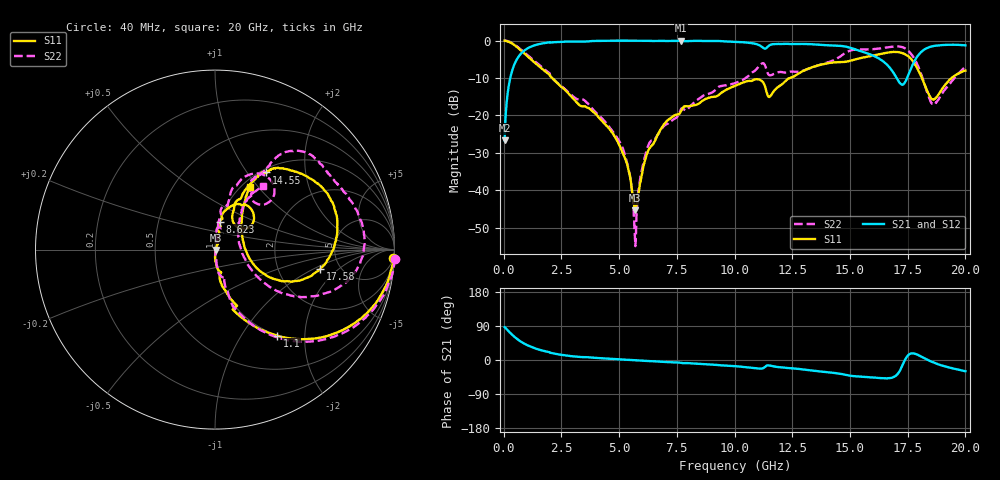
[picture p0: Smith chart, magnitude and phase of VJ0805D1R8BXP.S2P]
! VJ0805D1R8BXP
! DATE 10/29/2021  11:30
! CAPACITORS MOUNTED IN SERIES ON 25 MIL THICK MICROSTRIP SUBSTRATE
# GHz  S  MA  R  50.00
!  FREQ  S11M  S11A  S21M  S21A  S12M  S12A  S22M  S22A
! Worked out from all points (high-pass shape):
!   1601 points, 40 MHz to 20 GHz, reference 50 ohm
!   highest |S21| = 0.00 dB at 7.662 GHz (marker M1); lowest = -26.6 dB at 40 MHz (marker M2)
!   |S21| within 3 dB of the highest: 831 MHz to 15.55 GHz (14.72 GHz wide, 180 % of centre); 18.09 GHz to end of sweep
!   lowest |S11| = -45.3 dB at 5.704 GHz (marker M3), VSWR 1.01, Z = 50.5 - j0.143 ohm
!   |S11| at or under -10 dB: 2.098 GHz to 12.41 GHz (10.31 GHz wide, 142 % of centre); 18.12 GHz to 19.4 GHz (1.282 GHz wide, 6.84 % of centre)
!   |S22| runs from -54.9 to 0.0 dB; largest |S21 - S12| = 0.0054
!   S11 on the Smith chart (normalised r, x): 40 MHz: 5, -43; 1.1 GHz: 0.99, -1.46; 8.623 GHz: 1.00, +0.32; 14.55 GHz: 1.05, +1.23; 17.58 GHz: 3.53, -1.18; 20 GHz: 1.09, +0.90
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0.04  0.9948 -2.6  0.0466 86.9  0.04845 87.9  1.002 -3.0
0.202175  0.9678 -13.3  0.2306 76.5  0.2308 76.6  0.9792 -13.4
0.376825  0.9087 -23.8  0.4058 66.1  0.405 66.1  0.9218 -24.2
1.100375  0.5908 -54.1  0.8059 36.8  0.8061 36.8  0.613 -53.8
3.370825  0.1331 -75.7  0.9654 7.6  0.9644 7.6  0.1629 -70.7
5.10485  0.03464 -88.9  0.9979 1.4  0.9974 1.4  0.03957 -82.0
5.441675  0.01696 -81.6  0.9969 0.3  0.9959 0.2  0.0172 -79.2
5.70365  0.005406 -15.2  0.9961 -0.7  0.9963 -0.8  0.00179 8.1
6.140275  0.02647 64.8  0.9945 -2.3  0.9939 -2.4  0.02999 84.9
6.70165  0.05725 75.5  0.9915 -4.1  0.9909 -4.1  0.05684 81.3
7.662225  0.1108 83.0  0.9999 -7.4  0.9981 -7.5  0.1185 84.1
8.6228  0.158 80.9  0.9882 -10.8  0.9869 -10.9  0.1819 81.1
10.02  0.2484 71.1  0.9623 -16.2  0.9604 -16.4  0.2704 74.2
11.05542  0.3024 48.0  0.8717 -22.6  0.8708 -22.6  0.4504 66.4
11.52947  0.1779 52.5  0.8703 -14.6  0.8694 -14.7  0.343 49.7
13.35083  0.4394 60.7  0.8929 -27.8  0.8918 -27.9  0.4365 62.3
14.54842  0.5158 56.5  0.8502 -36.0  0.8498 -36.4  0.6043 56.6
16.68165  0.6941 28.2  0.4488 -48.2  0.4488 -48.3  0.8144 16.5
17.24302  0.6829 6.5  0.2575 -18.3  0.2572 -18.4  0.8221 -2.8
17.57985  0.5963 -10.4  0.3797 15.5  0.3789 15.5  0.7031 -18.5
18.6028  0.1642 12.4  0.844 -6.3  0.8432 -6.4  0.1402 9.7
20  0.3971 60.9  0.8631 -29.7  0.8624 -29.8  0.4447 52.7
